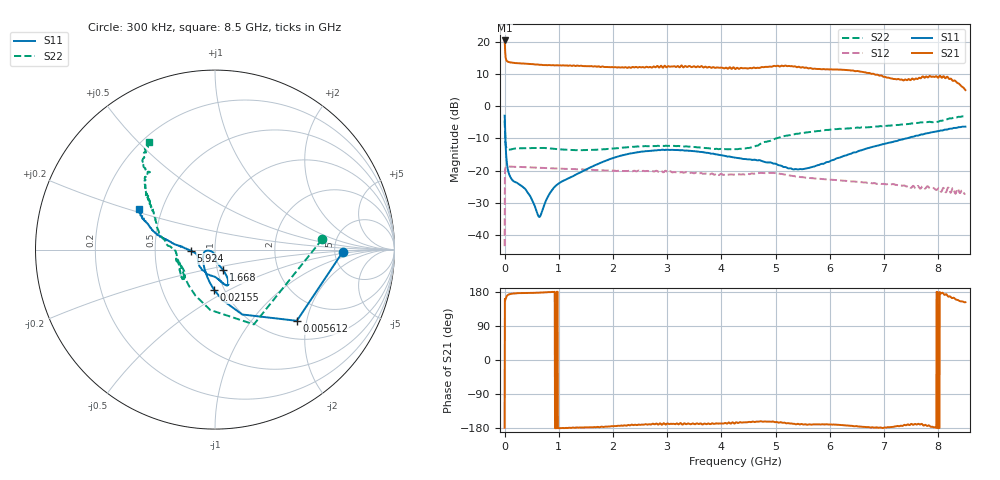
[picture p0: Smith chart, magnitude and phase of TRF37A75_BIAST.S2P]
!Agilent Technologies,E5071B,JP1KK00322,A.09.10
!Date: Mon Mar 03 16:32:35 2014
!Data & Calibration Information:
!Freq	S11:SOLT2(ON)	S21:SOLT2(ON)	S12:SOLT2(ON)	S22:SOLT2(ON)
# Hz S RI R 50
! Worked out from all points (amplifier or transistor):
!   1601 points, 300 kHz to 8.5 GHz, reference 50 ohm
!   highest |S21| = 20.4 dB at 300 kHz (marker M1)
!   |S21| within 3 dB of that: start of sweep to 9.552 MHz
!   unconditionally stable (mu >= 1): start of sweep to 2.048 MHz; 23.82 MHz to end of sweep
!   at 1.413 GHz: K = 1.29, MAG = 12.9 dB, |S12| = -19.7 dB
!   at 4.25 GHz: K = 1.61, MAG = 11.8 dB, |S12| = -21.2 dB
!   at 8.5 GHz: K = 2.58, MAG = 9.2 dB, |S12| = -27.3 dB
!   S11 on the Smith chart (normalised r, x): 300 kHz: 5.96, -0.26; 5.612 MHz: 1.40, -1.75; 21.55 MHz: 0.90, -0.42; 1.668 GHz: 1.06, -0.24; 5.924 GHz: 0.77, -0.01; 8.5 GHz: 0.37, +0.22
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300000  0.7132 -0.0106  -10.52 -0.2211  -0.00263 0.00613  0.5969 0.057
5612313  0.456 -0.3968  -8.586 2.9  0.0564 0.061  0.2165 -0.4166
2.154925e7  -0.00526 -0.2238  -5.323 1.659  0.1084 0.0296  -0.1438 -0.2043
5.342312e7  -0.0615 -0.0934  -4.892 0.7794  0.1145 0.0136  -0.1883 -0.0982
9.592162e7  -0.0672 -0.0483  -4.791 0.5219  0.1149 0.00933  -0.1994 -0.0696
6.430898e8  -0.012 -0.0147  -4.407 0.1627  0.1078 0.0228  -0.2155 -0.0638
9.299547e8  0.00483 -0.0563  -4.317 -0.0043  0.1021 0.0342  -0.205 -0.0711
1.418687e9  0.0264 -0.0916  -4.254 -0.1185  0.0902 0.0512  -0.1792 -0.1043
1.668366e9  0.0442 -0.1129  -4.173 -0.2012  0.0826 0.0586  -0.1717 -0.1213
2.837075e9  0.0732 -0.1947  -4.024 -0.6746  0.0431 0.0852  -0.1775 -0.1642
4.25015e9  0.0103 -0.1584  -3.704 -0.8585  -0.0152 0.0855  -0.2129 -0.0311
4.924814e9  -0.0744 -0.1092  -3.923 -1.218  -0.0364 0.0845  -0.2901 0.0618
5.211679e9  -0.0943 -0.0571  -4.083 -0.9555  -0.0371 0.0765  -0.3245 0.1297
5.668537e9  -0.1116 -0.0177  -3.779 -0.6254  -0.0471 0.0599  -0.3413 0.2094
5.923528e9  -0.133 -0.00697  -3.672 -0.6751  -0.0518 0.0515  -0.3563 0.2359
6.534444e9  -0.2015 0.0208  -3.476 -0.2689  -0.0585 0.0317  -0.3693 0.2769
7.086925e9  -0.2651 0.0527  -2.77 -0.1262  -0.0607 0.0131  -0.3847 0.3176
7.389727e9  -0.305 0.0708  -2.576 -0.3776  -0.0575 0.00517  -0.3907 0.3486
7.665967e9  -0.3448 0.1043  -2.693 -0.4666  -0.0522 -0.00456  -0.3911 0.4
8.06439e9  -0.3871 0.1601  -2.771 0.1661  -0.0448 -0.0173  -0.3878 0.4513
8.345943e9  -0.4179 0.2023  -2.164 0.835  -0.0434 -0.0262  -0.3873 0.5502
8.5e9  -0.4239 0.2273  -1.581 0.823  -0.0368 -0.0225  -0.3651 0.5987
